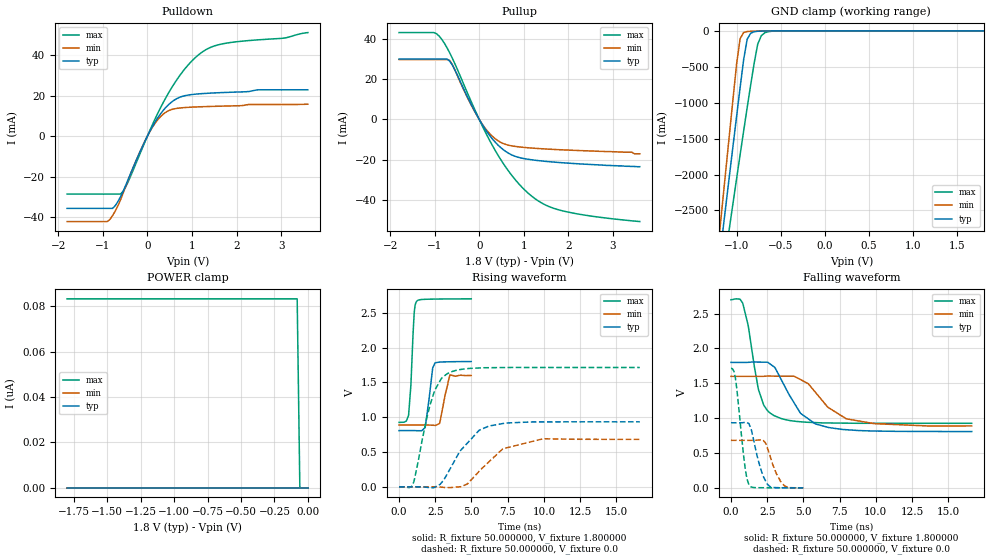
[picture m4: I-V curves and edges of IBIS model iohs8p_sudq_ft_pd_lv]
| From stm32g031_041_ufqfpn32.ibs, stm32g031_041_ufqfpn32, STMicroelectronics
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|   Model iohs8p_sudq_ft_pd_lv
[Model]  iohs8p_sudq_ft_pd_lv
Model_type I/O
Polarity   Non-Inverting
Enable   Active-Low
Vinl =   0.540000V
Vinh =   1.260000V
Vmeas =  0.900000V
Cref =   40.000000pF
Rref =   100.000000M
Vref =   0.0V
C_comp   1.984800pF   1.899400pF   2.077500pF
[Temperature Range]   25.000000   -40.000000   0.125000k
[Pullup Reference]   1.800000V   1.600000V   2.700000V
[Pulldown Reference]   0.0V   0.0V   0.0V
[POWER Clamp Reference]   1.800000V   1.600000V   2.700000V
[GND Clamp Reference]   0.0V   0.0V   0.0V
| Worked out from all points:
|   slope of the pulldown table from 0 to 0.27 V, typ, clamps not added: 26.4 ohm
|   slope of the pullup table from 0 to 0.27 V, typ, clamps not added: 30.1 ohm
|   GND clamp passes 1 mA (typ) near -0.60 V on its own axis
|   rising waveform, R_fixture 50.000000, V_fixture 1.800000: 20-80 % time 358ps typ, 426ps min, 254ps max; typ from 0.808 V to 1.8 V
|   rising waveform, R_fixture 50.000000, V_fixture 0.0: 20-80 % time 1.91ns typ, 2.02ns min, 1.14ns max; typ from 0 V to 0.933 V
|   falling waveform, R_fixture 50.000000, V_fixture 1.800000: 20-80 % time 1.88ns typ, 2.16ns min, 937ps max; typ from 1.8 V to 0.808 V
|   falling waveform, R_fixture 50.000000, V_fixture 0.0: 20-80 % time 697ps typ, 757ps min, 515ps max; typ from 0.933 V to 0 V
[Pulldown]
|Voltage   I(typ)   I(min)   I(max)
-1.8V     -35.64mA   -42.15mA   -28.59mA
-900mV    -35.64mA   -42.15mA   -28.59mA
-780mV    -35.64mA   -39.2mA    -28.59mA
-600mV    -29.83mA   -31.31mA   -28.52mA
-420mV    -20.8mA    -21.07mA   -21.98mA
60mV      2.604mA    2.459mA    3.062mA
240mV     9.303mA    8.31mA     11.61mA
480mV     15.67mA    12.64mA    21.52mA
720mV     19.18mA    13.91mA    29.74mA
960mV     20.46mA    14.3mA     36.27mA
1.44V     21.29mA    14.7mA     44.06mA
3.6V      22.91mA    15.79mA    51.15mA
[Pullup]
|Voltage   I(typ)   I(min)   I(max)
-1.8V     29.95mA    29.75mA    43.09mA
-1.02V    29.95mA    29.75mA    43.09mA
-900mV    29.95mA    29.75mA    41.34mA
-660mV    28.86mA    29.2mA     32.89mA
-60mV     2.392mA    2.26mA     2.893mA
300mV     -9.801mA   -8.48mA    -13.12mA
480mV     -13.91mA   -11.33mA   -19.82mA
720mV     -17.48mA   -13.04mA   -27.45mA
1.2V      -20.05mA   -14.2mA    -38.43mA
1.5V      -20.78mA   -14.63mA   -42.54mA
1.92V     -21.53mA   -15.1mA    -45.56mA
3.6V      -23.4mA    -17mA      -50.6mA
[GND_clamp]
|Voltage   I(typ)   I(min)   I(max)
-1.8V     -9.477A    -9.805A    -9.016A
-1.2V     -3.243A    -2.9A      -3.759A
-1.16V    -2.83A     -2.409A    -3.417A
-1.12V    -2.418A    -1.919A    -3.076A
-1.08V    -2.008A    -1.431A    -2.736A
-1V       -1.194A    -466mA     -2.061A
-960mV    -792.8mA   -108.7mA   -1.727A
-920mV    -402mA     -24.36mA   -1.396A
-880mV    -117.8mA   -9.2mA     -1.071A
-760mV    -5.909mA   -2.892mA   -183.8mA
-680mV    -2.407mA   -1.111mA   -26.63mA
1.8V      47.61uA    33.87uA    60.56uA
[POWER_clamp]
|Voltage   I(typ)   I(min)   I(max)
-1.8V     0A         0A         83.17nA
-80mV     0A         0A         83.17nA
-60mV     0A         0A         0A
0V        0A         0A         0A
[Ramp]
| variable   typ   min   max
dV/dt_r  0.56020/1.90925n   0.40837/2.01516n   1.02678/1.14258n
dV/dt_f  0.59489/1.87615n   0.42528/2.14494n   1.06359/0.93576n
R_load = 50.000000
[Rising Waveform]
R_fixture= 50.000000
V_fixture= 1.800000
V_fixture_min= 1.600000
V_fixture_max= 2.700000
|time   V(typ)   V(min)   V(max)
0s        807.9mV    888.7mV    925.8mV
660.7ps   808mV      888.7mV    1.029V
820.8ps   807.9mV    888.7mV    1.471V
1.051ns   807.6mV    888.7mV    2.508V
1.211ns   806.5mV    888.7mV    2.663V
1.802ns   851.7mV    888.1mV    2.692V
2.472ns   1.776V     882.7mV    2.696V
2.813ns   1.791V     917.4mV    2.696V
3.514ns   1.796V     1.608V     2.698V
4.985ns   1.799V     1.599V     2.699V
[Rising Waveform]
R_fixture= 50.000000
V_fixture= 0.0
V_fixture_min= 0.0
V_fixture_max= 0.0
|time   V(typ)   V(min)   V(max)
0s        60.06nV    530.2nV    51.3uV
1.001ns   18.18uV    -739.2nV   61.41mV
2.135ns   -11.66mV   63.26uV    1.173V
2.936ns   61.5mV     -4.204mV   1.56V
3.403ns   213.8mV    -10.31mV   1.632V
4.705ns   625.6mV    39.87mV    1.697V
6.206ns   872.9mV    359.3mV    1.711V
7.174ns   909.4mV    547.1mV    1.713V
9.943ns   932.7mV    690.1mV    1.714V
16.62ns   933.5mV    681.5mV    1.714V
[Falling Waveform]
R_fixture= 50.000000
V_fixture= 1.800000
V_fixture_min= 1.600000
V_fixture_max= 2.700000
|time   V(typ)   V(min)   V(max)
0s        1.799V     1.599V     2.699V
800.8ps   1.799V     1.599V     2.654V
1.201ns   1.8V       1.599V     2.316V
1.902ns   1.804V     1.599V     1.407V
2.269ns   1.803V     1.6V       1.185V
2.97ns    1.736V     1.602V     1.037V
4.805ns   1.069V     1.552V     947.8mV
5.839ns   916.2mV    1.368V     935.9mV
7.975ns   833.6mV    989.4mV    927.8mV
16.62ns   807.9mV    888.7mV    925.8mV
[Falling Waveform]
R_fixture= 50.000000
V_fixture= 0.0
V_fixture_min= 0.0
V_fixture_max= 0.0
|time   V(typ)   V(min)   V(max)
0s        933.5mV    681.5mV    1.714V
310.3ps   933.4mV    681.5mV    1.571V
981ps     939mV      681.5mV    281.4mV
1.221ns   925.1mV    681.4mV    56.09mV
1.411ns   829.7mV    681.2mV    11.77mV
2.032ns   283.4mV    687.1mV    1.933mV
2.503ns   54.95mV    579.6mV    1.186mV
3.143ns   3.27mV     200.5mV    692.2uV
3.684ns   1.1mV      29.71mV    431.9uV
4.985ns   60.06nV    530.2nV    51.3uV
